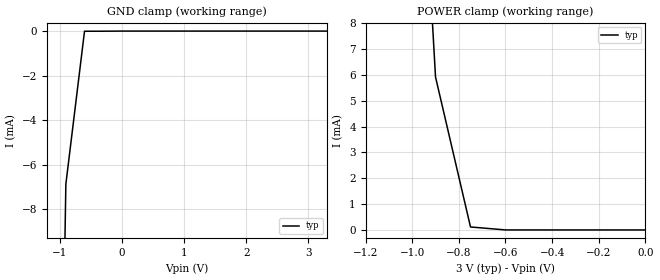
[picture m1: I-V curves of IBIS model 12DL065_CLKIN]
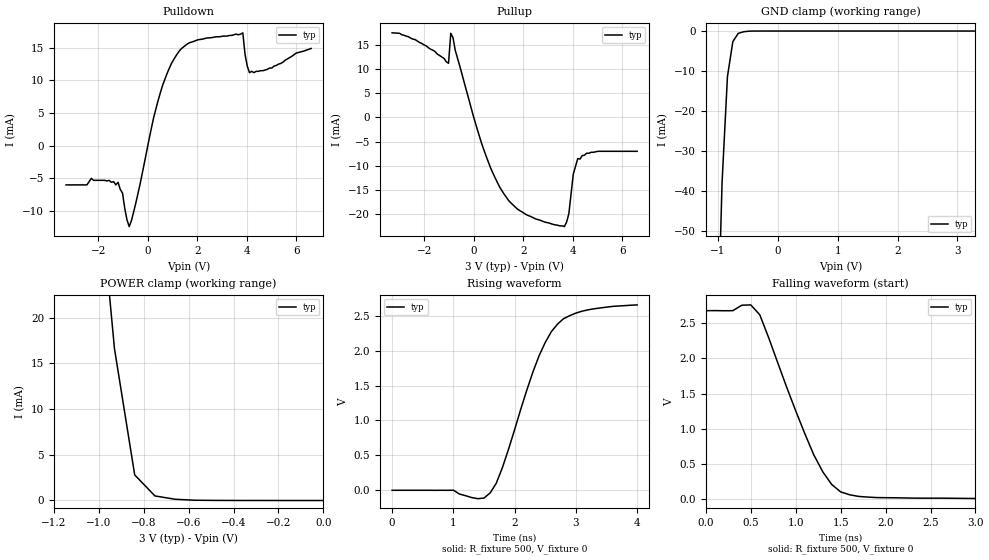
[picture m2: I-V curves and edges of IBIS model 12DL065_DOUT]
|   National Semiconductor Corporation
|   Data Conversion Products Group
|   IBIS Model of ADC12DL065
|   64 Pin TQFP Package
[IBIS Ver]   3.2
[File name]   adc12dl065.ibs
[File Rev]   1.1
[Date]   08/17/2006
[Source]   Spice/bench to Ibis Conversion
[Notes]   File created by RC,RL,IK
[Disclaimer]
(C) Copyright National Semiconductor Corporation 2005
   All rights reserved
   National Semiconductor Corporation hereby grants
the user of this IBIS model a non-exclusive, nontransferable
license to use this IBIS model under the following terms.
Before using this IBIS model, the user should read this
license.  If the user does not accept these terms,  the
IBIS model should be returned to National within 30 days.
   The user is granted this license only to use the
IBIS model and is not granted rights to sell, load, rent,
lease or license the IBIS model in whole or in part, or in
modified form to anyone other than user. User may modify
the IBIS model to suit its specific applications but rights
to derivative works and such modifications shall belong to
National.
   This IBIS model is provided on an "AS IS" basis and
National makes absolutely no warranty with respect to the
information contained herein.NATIONAL DISCLAIMS AND CUSTOMER
WAIVES ALL WARRANTIES, EXPRESS OR IMPLIED, INCLUDING
WARRANTIES OF MERCHANTABILITY OR FITNESS FOR A PARTICULAR
PURPOSE. The entire risk as to quality and performance is
with the Customer. ACCORDINGLY, IN NO EVENT SHALL THE
COMPANY BE LIABLE FOR ANY DAMAGES, WHETHER IN CONTRACT OR
TORT,INCLUDING ANY LOST PROFITS OR OTHER INCIDENTAL,
CONSEQUENTIAL, EXEMPLARY, OR PUNITIVE DAMAGES ARISING OUT
OF THE USE OR APPLICATION OF THE IBIS model provided in
this package.Further, National reserves the right to make
changes without notice to any product herein to improve
reliability, function, or design. National does not convey
any license under patent rights or any other intellectual
property rights, including those of third parties.
   National is not obligated to provide maintenance or support
for the licensed IBIS model.
Contact National at ATTN:DCS APPLICATIONS/IBIS MODELS.
2900 Semiconductor Drive, M/S D3-739, Santa Clara, CA 95052-8090
[Copyright]   Copyright 2005, National Semiconductor, All Rights Reserved
[Component]   ADC12DL065
[Manufacturer]  National Semiconductor Corp
[Package]
|   typ   min   max
R_pkg   277.0m   164.0m   357.0m
L_pkg   2.957nH   2.434n   3.554n
C_pkg   .136pF   .103pF   .262pF
[Pin]   signal_name   model_name   R_pin   L_pin   C_pin
1   VINB-   NC
2   VINB+   NC
3   AGND   GND   294.0m   3.011n   0.128p
4   VRMB   NC
5   VRPB   NC
6   VRNB   NC
7   VREF   NC
8   AGND   GND   257.0m   2.651n   0.112p
9   VA   POWER   257.0m   2.659n   0.111p
10   AGND   GND   256.0m   2.663n   0.119p
11   MULTIPLEX   NC
12   VRNA   NC
13   VRPA   NC
14   VRMA   NC
15   VINA+   NC
16   VINA-   NC
17   AGND   GND   357.0m   3.554n   0.244p
18   VA   POWER   336.0m   3.363n   0.145p
19   VA   POWER   318.0m   3.183n   0.130p
20   AGND   GND   195.0m   2.777n   0.140p
21   DFDCS   NC
22   OEA   NC
23   DRGND   GND   279.0m   2.837n   0.108p
24   DA0   12DL065_DOUT   276.0m   2.814n   0.107p
25   DA1   12DL065_DOUT   277.0m   2.815n   0.106p
26   DA2   12DL065_DOUT   178.0m   2.597n   0.123p
27   DA3   12DL065_DOUT   289.0m   2.918n   0.121p
28   DA4   12DL065_DOUT   296.0m   2.994n   0.108p
29   DA5   12DL065_DOUT   307.0m   3.097n   0.111p
30   VDR   POWER   322.0m   3.231n   0.123p
31   DRGND   GND   344.0m   3.401n   0.129p
32   DGND   GND   231.0m   3.281n   0.262p
33   VD   POWER   337.0m   3.398n   0.254p
34   DA6   12DL065_DOUT   314.0m   3.188n   0.144p
35   DA7   12DL065_DOUT   294.0m   3.011n   0.128p
36   DA8   12DL065_DOUT   276.0m   2.848n   0.123p
37   DA9   12DL065_DOUT   266.0m   2.744n   0.119p
38   DA10   12DL065_DOUT   164.0m   2.434n   0.120p
39   DA11   12DL065_DOUT   258.0m   2.645n   0.105p
40   DRGND   GND   257.0m   2.651n   0.112p
41   OEB   NC
42   DB0   12DL065_DOUT   256.0m   2.663n   0.119p
43   DB1   12DL065_DOUT   261.0m   2.701n   0.109p
44   DB2   12DL065_DOUT   171.0m   2.534n   0.130p
45   DB3   12DL065_DOUT   278.0m   2.861n   0.103p
46   DB4   12DL065_DOUT   295.0m   3.007n   0.110p
47   DB5   12DL065_DOUT   316.0m   3.172n   0.140p
48   VD   POWER   341.0m   3.386n   0.225p
49   DGND   GND   357.0m   3.554n   0.244p
50   DRGND   GND   336.0m   3.363n   0.145p
51   VDR   POWER   318.0m   3.183n   0.130p
52   DB6   12DL065_DOUT   195.0m   2.777n   0.140p
53   DB7   12DL065_DOUT   296.0m   2.956n   0.122p
54   DB8   12DL065_DOUT   286.0m   2.892n   0.122p
55   DB9   12DL065_DOUT   279.0m   2.837n   0.108p
56   DB10   12DL065_DOUT   276.0m   2.814n   0.107p
57   DB11   12DL065_DOUT   277.0m   2.815n   0.106p
58   DRGND   GND   178.0m   2.597n   0.123p
59   PD   NC
60   CLK   12DL065_CLKIN   296.0m   2.994n   0.108p
61   AGND   GND   307.0m   3.097n   0.111p
62   VA   POWER   322.0m   3.231n   0.123p
63   VA   POWER   344.0m   3.401n   0.129p
64   AGND   GND   231.0m   3.281n   0.262p
| Models and submodels in the file (2): 12DL065_CLKIN (Input), 12DL065_DOUT (3-state)
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|   Clock Input MODEL
[Model]   12DL065_CLKIN
Model_type Input
Vinh=2.0
Vinl=1.0
|   TYP   MIN   MAX
C_comp   0.1p   0.1p   0.1p
[Temperature Range] 27   NA   NA
[Voltage Range]   3.0   NA   NA
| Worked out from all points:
|   POWER clamp passes 1 mA (typ) near -0.77 V on its own axis
[GND Clamp]
|V(groundclamp)   I(typ)   I(min)   I(max)
-3.3V     -480mA     NA         NA
-1.2V     -57.8mA    NA         NA
-900mV    -6.88mA    NA         NA
-600mV    -7.06uA    NA         NA
3.3V      0A         NA         NA
[POWER Clamp]
|V(table)   I(typ)   I(min)   I(max)
-3.3V     529mA      NA         NA
-1.05V    29.8mA     NA         NA
-900mV    5.92mA     NA         NA
-750mV    116uA      NA         NA
-600mV    1.47uA     NA         NA
0V        0A         NA         NA
|   Driver Output MODEL
[Model]   12DL065_DOUT
Model_type 3-state
Polarity Non-Inverting
|   TYP   MIN   MAX
C_comp   0.1p   0.1p   0.1p
[Temperature Range] 27   NA   NA
[Voltage Range]   3.0   NA   NA
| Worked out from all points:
|   slope of the pulldown table from 0 to 0.45 V, typ, clamps not added: 61.1 ohm
|   slope of the pullup table from 0 to 0.45 V, typ, clamps not added: 61.6 ohm
|   GND clamp passes 1 mA (typ) near -0.68 V on its own axis
|   POWER clamp passes 1 mA (typ) near -0.77 V on its own axis
|   falling waveform, R_fixture 500, V_fixture 0: 20-80 % time 496ps typ, NA min, NA max; typ from 2.68 V to 0.002 V
|   rising waveform, R_fixture 500, V_fixture 0: 20-80 % time 625ps typ, NA min, NA max; typ from 0 V to 2.65 V
[GND Clamp]
|V(groundclamp)   I(typ)   I(min)   I(max)
-3.3V     -1.889A    NA         NA
-1.02V    -87.1mA    NA         NA
-930mV    -37.9mA    NA         NA
-840mV    -11.4mA    NA         NA
-750mV    -2.66mA    NA         NA
-660mV    -586uA     NA         NA
-570mV    -186uA     NA         NA
-390mV    -2.69uA    NA         NA
3.3V      0A         NA         NA
[POWER Clamp]
|V(table)   I(typ)   I(min)   I(max)
-3.3V     783mA      NA         NA
-1.02V    40.3mA     NA         NA
-930mV    16.6mA     NA         NA
-840mV    2.8mA      NA         NA
-750mV    499uA      NA         NA
-660mV    134uA      NA         NA
-570mV    26.8uA     NA         NA
0V        0A         NA         NA
[Pullup]
|Vtable   I(typ)   I(min)   I(max)
-3.3V     17.5mA     NA         NA
-1.02V    11.2mA     NA         NA
-930mV    17.4mA     NA         NA
60mV      -1.056mA   NA         NA
690mV     -10.57mA   NA         NA
1.41V     -17.19mA   NA         NA
2.13V     -20.12mA   NA         NA
3.66V     -22.56mA   NA         NA
3.84V     -19.9mA    NA         NA
4.02V     -11.72mA   NA         NA
4.2V      -8.5mA     NA         NA
6.6V      -7mA       NA         NA
[Pulldown]
|V(pulldown)   I(typ)   I(min)   I(max)
-3.3V     -6mA       NA         NA
-1.2V     -5.6mA     NA         NA
-1.02V    -7.24mA    NA         NA
-750mV    -12.39mA   NA         NA
-480mV    -8.731mA   NA         NA
420mV     6.957mA    NA         NA
870mV     11.87mA    NA         NA
1.32V     14.73mA    NA         NA
3.84V     17.3mA     NA         NA
4.02V     12.2mA     NA         NA
4.29V     11.2mA     NA         NA
6.6V      14.9mA     NA         NA
[Ramp]
|   TYP   MIN   MAX
dV/dt_r   2.18/5.5E-10   NA   NA
dV/dt_f   2.18/7.0E-10   NA   NA
R_load=500
[Falling Waveform]
R_fixture=500
V_fixture=0
|Time   V(typ)   V(min)   V(max)
0s        2.681V     NA         NA
300ps     2.681V     NA         NA
500ps     2.763V     NA         NA
600ps     2.622V     NA         NA
1ns       1.253V     NA         NA
1.2ns     629.7mV    NA         NA
1.4ns     204.9mV    NA         NA
1.5ns     98.64mV    NA         NA
1.9ns     17.85mV    NA         NA
4ns       1.872mV    NA         NA
[Rising Waveform]
R_fixture=500
V_fixture=0
|Time   V(typ)   V(min)   V(max)
0s        72.64uV    NA         NA
1ns       1.522mV    NA         NA
1.5ns     -111.1mV   NA         NA
1.7ns     100.6mV    NA         NA
1.9ns     586.5mV    NA         NA
2.3ns     1.698V     NA         NA
2.6ns     2.273V     NA         NA
2.8ns     2.459V     NA         NA
3ns       2.538V     NA         NA
4ns       2.655V     NA         NA
